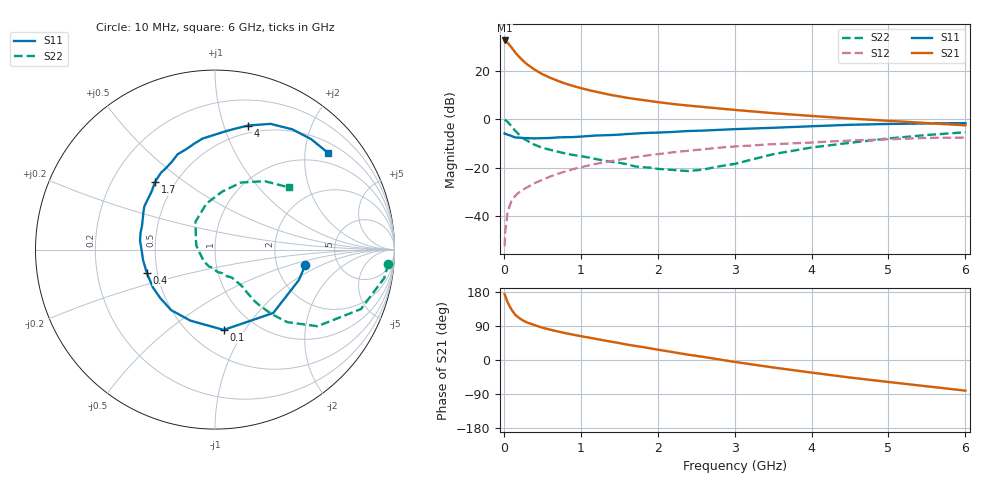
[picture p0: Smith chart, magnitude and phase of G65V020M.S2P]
! SIEMENS Small Signal Semiconductors
! BFG193
! Si NPN RF Bipolar Junction Transistor in SOT223
! VCE = 5 V  IC = 20 mA
! Common Emitter S-Parameters:  August  1996
# GHz  S  MA  R  50
!  f  S11  S21  S12  S22
! GHz  MAG  ANG  MAG  ANG  MAG  ANG  MAG  ANG
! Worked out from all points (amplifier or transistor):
!   36 points, 10 MHz to 6 GHz, reference 50 ohm
!   highest |S21| = 32.5 dB at 10 MHz (marker M1)
!   |S21| within 3 dB of that: start of sweep to 102 MHz
!   unconditionally stable (mu >= 1): 706.9 MHz to 2.42 GHz
!   at 250 MHz: K = 0.74, MSG = 26.6 dB, |S12| = -29.1 dB
!   at 1.4 GHz: K = 1.05, MAG = 12.2 dB, |S12| = -17.3 dB
!   at 6 GHz: K = 0.88, MSG = 2.5 dB, |S12| = -7.6 dB
!   S11 on the Smith chart (normalised r, x): 10 MHz: 2.89, -0.69; 100 MHz: 0.72, -0.81; 400 MHz: 0.44, -0.13; 1.7 GHz: 0.39, +0.39; 4 GHz: 0.43, +1.20; 6 GHz: 0.73, +2.52
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0.01  0.51 -10.0  42.06 173.5  0.0024 86.8  0.9694 -4.7
0.02  0.4969 -20.1  41.35 168.2  0.0052 79.4  0.9559 -9.6
0.05  0.4796 -47.4  37.68 151.4  0.0125 72.8  0.8778 -22.2
0.1  0.45 -83.8  30.07 132.9  0.0207 64.9  0.7126 -36.8
0.15  0.4189 -109.1  23.57 118.9  0.0264 60.0  0.5705 -45.1
0.2  0.4164 -126.0  19.22 110.7  0.0311 58.9  0.4785 -48.7
0.25  0.4072 -138.7  15.99 104.2  0.0352 58.4  0.4064 -51.1
0.3  0.4051 -148.6  13.65 99.2  0.0391 59.4  0.3614 -52.5
0.4  0.4014 -161.3  10.54 92.0  0.0478 60.2  0.2963 -53.3
0.5  0.4053 -171.9  8.503 85.3  0.056 60.5  0.2579 -53.5
0.6  0.4091 -179.8  7.18 80.2  0.0656 60.9  0.2335 -54.5
0.7  0.4204 173.3  6.191 75.3  0.0743 60.4  0.214 -56.3
0.9  0.4274 162.2  4.846 66.8  0.0933 58.0  0.1829 -58.9
1.1  0.4482 153.1  3.992 59.3  0.1108 55.7  0.1621 -65.9
1.4  0.4714 141.0  3.142 48.2  0.1366 50.5  0.132 -77.2
1.7  0.5039 131.6  2.619 37.4  0.1641 45.2  0.1065 -91.6
2.2  0.5455 116.1  2.054 20.7  0.2073 34.5  0.0896 -133.8
3.5  0.6643 84.4  1.331 -19.7  0.3045 4.6  0.1895 125.0
4  0.7144 75.3  1.167 -33.2  0.3303 -5.0  0.2604 100.7
4.5  0.7658 66.2  1.03 -46.3  0.3631 -15.2  0.3255 83.0
5.5  0.8158 49.0  0.831 -69.4  0.4116 -38.7  0.4716 53.9
6  0.8288 40.6  0.747 -80.9  0.4188 -52.3  0.5372 40.2
